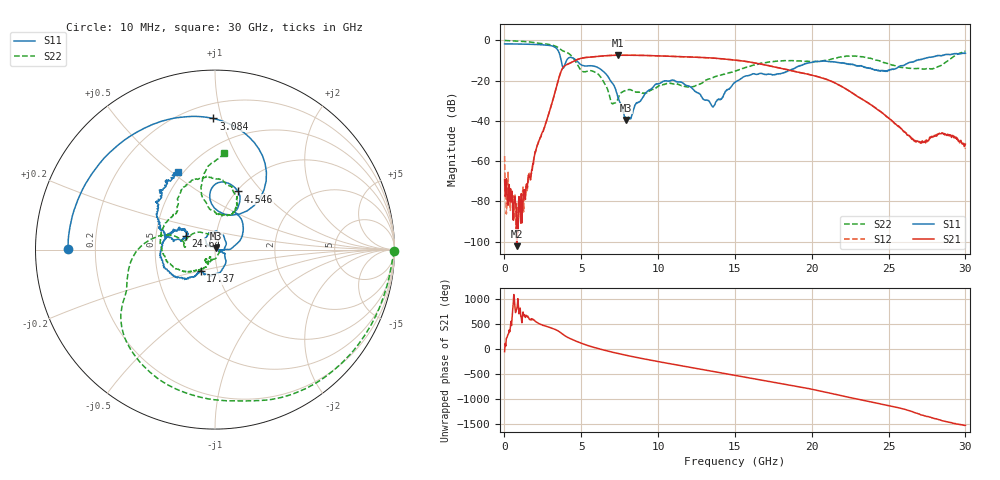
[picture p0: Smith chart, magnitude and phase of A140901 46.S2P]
!  2-Port S-parameters saved by WinCal
! VAR MeasName=S-Parameters (CALIBRATED_DATA) read from VNA (N5244A)
! VAR MeasDate=11/3/2014 9:34:11 AM
! VAR NAME=A140901 46
! VAR FILENAME=A140901 46.S2P
! VAR DATE=11/3/2014 9:34:11 AM
! VAR PHYS_PORTS=1,2
# Hz S RI R 50
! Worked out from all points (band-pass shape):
!   801 points, 10 MHz to 30 GHz, reference 50 ohm
!   highest |S21| = -7.36 dB at 7.395 GHz (marker M1); lowest = -102.2 dB at 797.2 MHz (marker M2)
!   |S21| within 3 dB of the highest: 4.508 GHz to 15.61 GHz (11.1 GHz wide, 110 % of centre)
!   lowest |S11| = -39.6 dB at 7.92 GHz (marker M3), VSWR 1.02, Z = 50.4 + j0.972 ohm
!   |S11| at or under -10 dB: 3.693 GHz to 4.042 GHz (349.2 MHz wide, 9.03 % of centre); 4.688 GHz to 26.77 GHz (22.08 GHz wide, 140 % of centre); 26.78604 GHz to 26.82225 GHz (36.21 MHz wide, 0.135 % of centre)
!   |S22| runs from -31.5 to 0.0 dB; largest |S21 - S12| = 0.0028
!   S11 on the Smith chart (normalised r, x): 10 MHz: 0.10, +0.00; 3.084 GHz: 0.30, +0.94; 4.546 GHz: 1.02, +0.75; 17.37 GHz: 0.83, -0.20; 24.64 GHz: 0.71, +0.11; 30 GHz: 0.47, +0.52
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1e7  -0.8189 0.00316  0.000204 -0.000285  -0.00075 0.00109  0.9963 -0.00835
1.974375e8  -0.8166 0.0644  -1.62e-05 -9.16e-05  4.77e-05 -9.67e-05  0.9745 -0.1313
7.972375e8  -0.7725 0.2555  2.06e-06 7.45e-06  -6.61e-05 -2.47e-05  0.8377 -0.4727
1.397038e9  -0.6774 0.434  0.00015 -0.000157  0.000105 -0.000218  0.5798 -0.7329
3.083975e9  -0.00907 0.7305  0.0156 0.0219  0.0157 0.0219  -0.3807 -0.6657
3.75875e9  0.1356 0.1977  0.1013 -0.1681  0.1012 -0.1672  -0.5001 -0.2543
4.545988e9  0.1289 0.3242  -0.3031 0.0564  -0.3032 0.056  -0.3274 0.0704
5.033325e9  0.1129 0.2145  -0.12 0.342  -0.1204 0.3418  -0.1707 0.0353
6.15795e9  0.156 0.1308  0.404 0.0133  0.4035 0.0138  -0.0979 0.0961
7.020162e9  0.0875 0.00308  0.1759 -0.3866  0.1767 -0.3864  0.0249 0.0103
7.395038e9  0.0371 -0.00288  -0.017 -0.4282  -0.0163 -0.428  0.0135 -0.034
7.919862e9  0.00422 0.00964  -0.26 -0.3392  -0.2591 -0.3394  -0.018 -0.0549
1.001916e10  -0.0527 0.0657  -0.1129 0.3983  -0.1125 0.3972  -0.0289 -0.0676
1.204349e10  0.0632 0.0353  0.3866 -0.0307  0.3859 -0.0302  -0.0427 -0.0546
1.358048e10  0.0203 -0.00884  0.015 -0.3628  0.0155 -0.3626  -0.061 -0.1025
1.5005e10  0.0611 -0.0662  -0.3145 -0.0798  -0.3142 -0.0804  -0.1228 -0.1205
1.736671e10  -0.0799 -0.1182  0.1024 0.2032  0.1014 0.2043  -0.2937 -0.00855
2.002832e10  -0.2616 -0.1174  0.00893 -0.1358  0.00909 -0.1366  -0.2156 0.2009
2.463929e10  -0.1622 0.0776  0.0133 -0.0077  0.0133 -0.00771  0.1199 0.2595
2.501416e10  -0.1648 0.064  0.00686 -0.00944  0.00697 -0.00934  0.1187 0.2343
2.677608e10  -0.2995 0.1041  -0.00296 0.00099  -0.00281 0.00102  0.0565 0.1917
3e10  -0.2086 0.4323  0.000163 -0.00263  -2.6e-05 -0.00202  0.0519 0.5362
